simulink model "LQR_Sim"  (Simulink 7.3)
settings: Solver=ode45  StartTime=0.0  StopTime=20  RelTol=1e-3
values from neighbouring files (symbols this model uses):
  calfa = cosd(alfa)    [LQR_Design.m]
  d2r = pi/180    (= 0.0174532925199)    [LQR_Design.m]    (also in init.m; pl.m)
  ge = 32.174    [LQR_Design.m]
  r2d = 180/pi    (= 57.2957795131)    [LQR_Design.m]    (also in init.m; pl.m)
  salfa = sind(alfa)    [LQR_Design.m]
  Thet0 = 3    [LQR_Design.m]
  V0 = 400    [LQR_Design.m]
undefined symbols (not defined in the file or in its folder): As, Av2, Avl, Avp, Bs, Bv2, Bvl, Bvp, Cs, Cv2, Cvl, Cvp, Ds, Dv2, Dvl, Dvp, Kpr, Kq

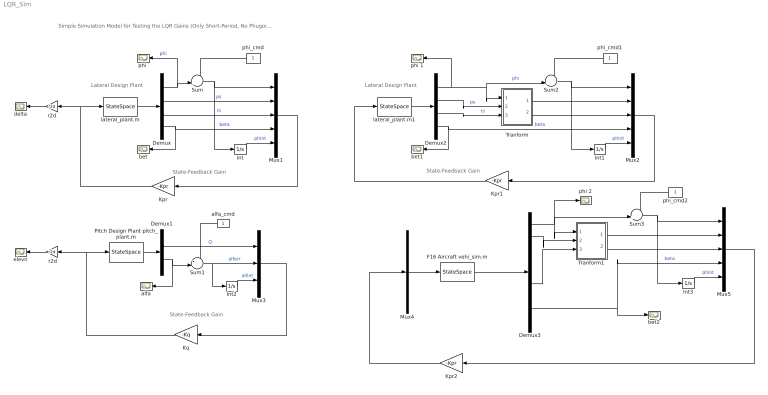
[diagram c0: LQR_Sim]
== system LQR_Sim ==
  note: Simple Simulation Model for Testing the LQR Gains (Only Short-Period, No Phugoid)
  note: Lateral Design Plant
  note: State-Feedback Gain
  note: State-Feedback Gain
  note: Lateral Design Plant
  note: State-Feedback Gain
  " r2d" : Gain  Gain=r2d  ParameterDataType=fixdt(1, 16)  ParameterScaling=2^0  OutDataType=fixdt(1, 16)  OutScaling=2^0
  Demux : Demux
  Demux1 : Demux  Outputs=2
  Demux2 : Demux
  Demux3 : Demux  Outputs=[1 1 1 1 1 1 1 1 6]
  F16 Aircraft vehi_sim.m : StateSpace  A=As  B=Bs  C=Cs  D=Ds
  Int{,1..3} (4 alike) : Integrator
  Kpr : Gain  Gain=-Kpr  Multiplication=Matrix(K*u)  ParameterDataType=fixdt(1, 16)  ParameterScaling=2^0  OutDataType=fixdt(1, 16)  OutScaling=2^0
  Kpr1 : Gain  Gain=-Kpr  Multiplication=Matrix(K*u)  ParameterDataType=fixdt(1, 16)  ParameterScaling=2^0  OutDataType=fixdt(1, 16)  OutScaling=2^0
  Kpr2 : Gain  Gain=-Kpr  Multiplication=Matrix(K*u)  ParameterDataType=fixdt(1, 16)  ParameterScaling=2^0  OutDataType=fixdt(1, 16)  OutScaling=2^0
  Kq : Gain  Gain=-Kq  Multiplication=Matrix(K*u)  ParameterDataType=fixdt(1, 16)  ParameterScaling=2^0  OutDataType=fixdt(1, 16)  OutScaling=2^0
  Mux1 : Mux  Inputs=5
  Mux2 : Mux  Inputs=5
  Mux3 : Mux  Inputs=3
  Mux4 : Mux  Inputs=[1, 2, 1]
  Mux5 : Mux  Inputs=5
  Pitch Design Plant pitch_plant.m : StateSpace  A=Avp  B=Bvp  C=Cvp  D=Dvp
  Sum{,1..3} (4 alike) : Sum  Inputs=-+|  OutDataType=fixdt(1, 16)  OutScaling=2^0
  Tranform : Subsystem
  Tranform1 : Subsystem
  alfa : Scope
  alfa_cmd : Constant  OutDataType=fixdt(1, 16)  OutScaling=2^0
  bet : Scope
  bet1 : Scope
  bet2 : Scope
  delta : Scope
  elevn : Scope
  lateral_plant.m : StateSpace  A=Avl  B=Bvl  C=Cvl  D=Dvl
  lateral_plant.m1 : StateSpace  A=Av2  B=Bv2  C=Cv2  D=Dv2
  "phi " : Scope
  phi 1 : Scope
  phi 2 : Scope
  phi_cmd : Constant  OutDataType=fixdt(1, 16)  OutScaling=2^0
  phi_cmd1 : Constant  OutDataType=fixdt(1, 16)  OutScaling=2^0
  phi_cmd2 : Constant  OutDataType=fixdt(1, 16)  OutScaling=2^0
  r2d : Gain  Gain=r2d  ParameterDataType=fixdt(1, 16)  ParameterScaling=2^0  OutDataType=fixdt(1, 16)  OutScaling=2^0
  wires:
  Kpr/1 -> lateral_plant.m/1, r2d/1
  lateral_plant.m/1 -> Demux/1
  Demux/2 -> Mux1/2  "ps"
  Demux/3 -> Mux1/3  "rs"
  Demux/4 -> Mux1/4, bet/1  "beta"
  Int/1 -> Mux1/5  "phint"
  Demux/1 -> Sum/2, "phi "/1  "phi"
  Sum/1 -> Mux1/1, Int/1
  phi_cmd/1 -> Sum/1
  Mux1/1 -> Kpr/1
  r2d/1 -> delta/1
  Pitch Design Plant pitch_plant.m/1 -> Demux1/1
  Kq/1 -> Pitch Design Plant pitch_plant.m/1, " r2d"/1
  " r2d"/1 -> elevn/1
  Mux3/1 -> Kq/1
  Demux1/1 -> Mux3/1  "Q"
  Int2/1 -> Mux3/3  "alfint"
  Demux1/2 -> Sum1/2, alfa/1
  Sum1/1 -> Mux3/2, Int2/1  "alferr"
  alfa_cmd/1 -> Sum1/1
  Kpr1/1 -> lateral_plant.m1/1
  lateral_plant.m1/1 -> Demux2/1
  Demux2/4 -> bet1/1, Mux2/4  "beta"
  Int1/1 -> Mux2/5  "phint"
  Demux2/1 -> phi 1/1, Sum2/2, Tranform/1(phi)  "phi"
  Sum2/1 -> Mux2/1, Int1/1
  phi_cmd1/1 -> Sum2/1
  Mux2/1 -> Kpr1/1
  Tranform/1(p_s) -> Mux2/2
  Tranform/2(r_s) -> Mux2/3
  Demux2/3 -> Tranform/3(r_b)  "rs"
  Demux2/2 -> Tranform/2(p_b)  "ps"
  Mux4/1 -> F16 Aircraft vehi_sim.m/1
  Kpr2/1 -> Mux4/2
  F16 Aircraft vehi_sim.m/1 -> Demux3/1
  Int3/1 -> Mux5/5  "phint"
  Sum3/1 -> Mux5/1, Int3/1
  phi_cmd2/1 -> Sum3/1
  Demux3/1 -> Sum3/2, Tranform1/1(phi), phi 2/1
  Demux3/2 -> Tranform1/2(p_b)
  Demux3/6 -> Tranform1/3(r_b)
  Demux3/8 -> Mux5/4, bet2/1  "beta"
  Tranform1/1(p_s) -> Mux5/2
  Tranform1/2(r_s) -> Mux5/3
  Mux5/1 -> Kpr2/1

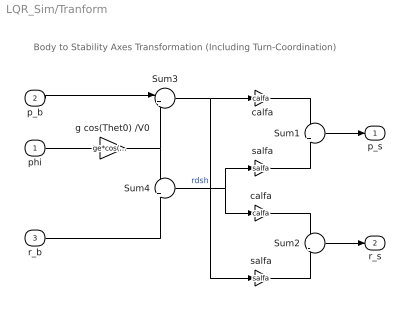
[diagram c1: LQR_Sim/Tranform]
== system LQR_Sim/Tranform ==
  note: Body to Stability Axes Transformation (Including Turn-Coordination)
  phi : Inport  OutDataType=sfix(16)  OutScaling=2^0
  p_b : Inport  Port=2  OutDataType=sfix(16)  OutScaling=2^0
  r_b : Inport  Port=3  OutDataType=sfix(16)  OutScaling=2^0
  Sum1 : Sum  Inputs=+|+  OutDataType=sfix(16)  OutScaling=2^0
  Sum2 : Sum  Inputs=+|-  OutDataType=sfix(16)  OutScaling=2^0
  Sum3 : Sum  Inputs=|++  OutDataType=sfix(16)  OutScaling=2^0
  Sum4 : Sum  Inputs=-|+  OutDataType=sfix(16)  OutScaling=2^0
  calfa : Gain  Gain=calfa  ParameterDataType=sfix(16)  ParameterScaling=2^0  OutDataType=sfix(16)  OutScaling=2^0
  "calfa " : Gain  Gain=calfa  ParameterDataType=sfix(16)  ParameterScaling=2^0  OutDataType=sfix(16)  OutScaling=2^0
  g cos(Thet0) /V0 : Gain  Gain=ge*cos(Thet0*d2r)/V0  ParameterDataType=sfix(16)  ParameterScaling=2^0  OutDataType=sfix(16)  OutScaling=2^0
  salfa : Gain  Gain=salfa  ParameterDataType=sfix(16)  ParameterScaling=2^0  OutDataType=sfix(16)  OutScaling=2^0
  "salfa " : Gain  Gain=salfa  ParameterDataType=sfix(16)  ParameterScaling=2^0  OutDataType=sfix(16)  OutScaling=2^0
  p_s : Outport  OutDataType=sfix(16)  OutScaling=2^0
  r_s : Outport  Port=2  OutDataType=sfix(16)  OutScaling=2^0
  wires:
  "salfa "/1 -> Sum2/2
  "calfa "/1 -> Sum2/1
  salfa/1 -> Sum1/2
  calfa/1 -> Sum1/1
  Sum3/1 -> calfa/1, "salfa "/1
  Sum4/1 -> salfa/1, "calfa "/1  "rdsh"
  phi/1 -> g cos(Thet0) /V0/1
  p_b/1 -> Sum3/1
  Sum1/1 -> p_s/1
  Sum2/1 -> r_s/1
  r_b/1 -> Sum4/2
  g cos(Thet0) /V0/1 -> Sum4/1, Sum3/2

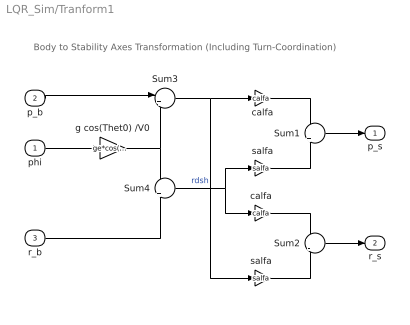
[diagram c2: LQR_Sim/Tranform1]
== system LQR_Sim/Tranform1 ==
  note: Body to Stability Axes Transformation (Including Turn-Coordination)
  phi : Inport  OutDataType=sfix(16)  OutScaling=2^0
  p_b : Inport  Port=2  OutDataType=sfix(16)  OutScaling=2^0
  r_b : Inport  Port=3  OutDataType=sfix(16)  OutScaling=2^0
  Sum1 : Sum  Inputs=+|+  OutDataType=sfix(16)  OutScaling=2^0
  Sum2 : Sum  Inputs=+|-  OutDataType=sfix(16)  OutScaling=2^0
  Sum3 : Sum  Inputs=|++  OutDataType=sfix(16)  OutScaling=2^0
  Sum4 : Sum  Inputs=-|+  OutDataType=sfix(16)  OutScaling=2^0
  calfa : Gain  Gain=calfa  ParameterDataType=sfix(16)  ParameterScaling=2^0  OutDataType=sfix(16)  OutScaling=2^0
  "calfa " : Gain  Gain=calfa  ParameterDataType=sfix(16)  ParameterScaling=2^0  OutDataType=sfix(16)  OutScaling=2^0
  g cos(Thet0) /V0 : Gain  Gain=ge*cos(Thet0*d2r)/V0  ParameterDataType=sfix(16)  ParameterScaling=2^0  OutDataType=sfix(16)  OutScaling=2^0
  salfa : Gain  Gain=salfa  ParameterDataType=sfix(16)  ParameterScaling=2^0  OutDataType=sfix(16)  OutScaling=2^0
  "salfa " : Gain  Gain=salfa  ParameterDataType=sfix(16)  ParameterScaling=2^0  OutDataType=sfix(16)  OutScaling=2^0
  p_s : Outport  OutDataType=sfix(16)  OutScaling=2^0
  r_s : Outport  Port=2  OutDataType=sfix(16)  OutScaling=2^0
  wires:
  "salfa "/1 -> Sum2/2
  "calfa "/1 -> Sum2/1
  salfa/1 -> Sum1/2
  calfa/1 -> Sum1/1
  Sum3/1 -> calfa/1, "salfa "/1
  Sum4/1 -> salfa/1, "calfa "/1  "rdsh"
  phi/1 -> g cos(Thet0) /V0/1
  p_b/1 -> Sum3/1
  Sum1/1 -> p_s/1
  Sum2/1 -> r_s/1
  r_b/1 -> Sum4/2
  g cos(Thet0) /V0/1 -> Sum4/1, Sum3/2
